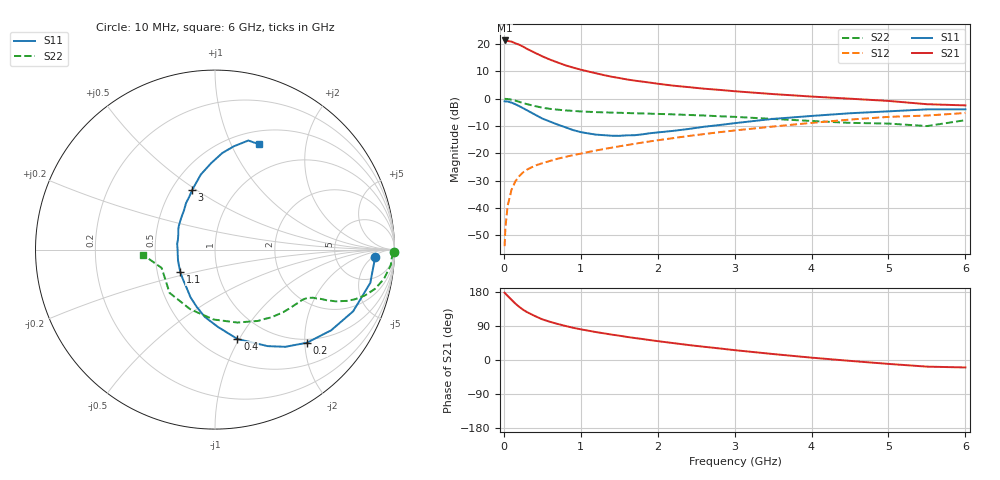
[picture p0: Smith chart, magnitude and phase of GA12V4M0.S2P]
! Infineon Technologies  Discrete & RF Semiconductors
! BF775
! Si NPN RF Bipolar Junction Transistor in SOT23
! VCE = 12 V  IC = 4 mA
! Common Emitter S-Parameters:  May  1996
# GHz  S  MA  R  50
!  f  S11  S21  S12  S22
! GHz  MAG  ANG  MAG  ANG  MAG  ANG  MAG  ANG
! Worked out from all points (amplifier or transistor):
!   36 points, 10 MHz to 6 GHz, reference 50 ohm
!   highest |S21| = 21.3 dB at 10 MHz (marker M1)
!   |S21| within 3 dB of that: start of sweep to 296.1 MHz
!   unconditionally stable (mu >= 1): 947.4 MHz to 2.929 GHz
!   at 250 MHz: K = 0.42, MSG = 23.0 dB, |S12| = -27.0 dB
!   at 1.4 GHz: K = 1.10, MAG = 11.1 dB, |S12| = -18.0 dB
!   at 6 GHz: K = 0.88, MSG = 1.4 dB, |S12| = -5.3 dB
!   S11 on the Smith chart (normalised r, x): 10 MHz: 15, -6; 200 MHz: 0.92, -2.04; 400 MHz: 0.73, -0.98; 1.1 GHz: 0.66, -0.18; 3 GHz: 0.63, +0.48; 6 GHz: 0.65, +1.28
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0.01  0.8922 -2.5  11.57 177.5  0.002 82.4  0.9948 -0.9
0.02  0.8892 -4.9  11.28 175.2  0.0043 84.3  0.9876 -2.0
0.05  0.8849 -12.1  11.33 169.0  0.0111 82.3  0.983 -5.1
0.1  0.8428 -24.1  11.03 158.9  0.0215 77.5  0.9549 -9.9
0.15  0.788 -34.8  10.25 148.8  0.0307 70.7  0.9177 -13.8
0.2  0.7288 -45.4  9.684 140.3  0.0382 67.2  0.8736 -17.0
0.25  0.6686 -54.1  8.926 132.7  0.0447 63.5  0.83 -19.4
0.3  0.6125 -61.4  8.134 126.5  0.0501 61.2  0.793 -21.1
0.4  0.5136 -75.9  6.94 116.4  0.059 58.2  0.7321 -23.2
0.5  0.4318 -87.7  5.927 107.3  0.0658 56.8  0.682 -24.4
0.6  0.3799 -98.5  5.171 100.8  0.0724 56.3  0.6494 -25.0
0.7  0.335 -107.7  4.574 95.1  0.0795 56.1  0.6275 -25.7
0.9  0.2658 -126.4  3.691 85.1  0.0926 56.6  0.5954 -26.8
1.1  0.2306 -146.7  3.126 77.3  0.1056 57.9  0.5739 -28.4
1.3  0.2144 -164.0  2.691 70.4  0.1197 58.1  0.5598 -30.2
1.6  0.213 171.5  2.24 60.9  0.1413 58.2  0.5446 -33.8
2.2  0.2568 137.5  1.726 44.7  0.1892 56.9  0.5153 -42.7
3  0.3555 111.0  1.364 26.0  0.2613 52.0  0.4638 -59.0
3.5  0.4257 100.7  1.21 15.7  0.3086 47.3  0.4249 -73.0
4.5  0.5395 85.7  0.996 -2.3  0.4134 36.1  0.3598 -112.5
5.5  0.6354 73.0  0.79 -17.5  0.4903 20.4  0.3143 -161.0
6  0.636 67.4  0.751 -19.7  0.5452 16.0  0.4034 -176.1
